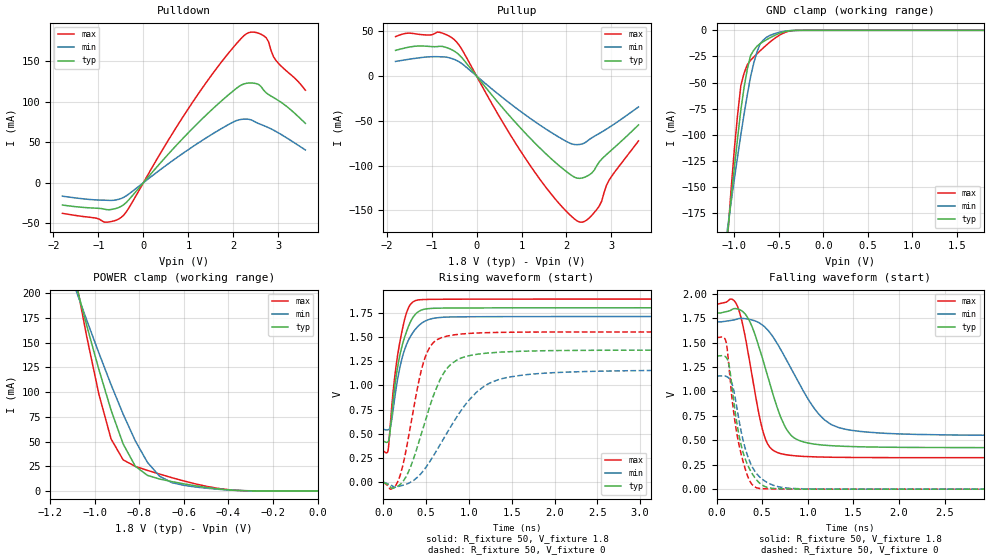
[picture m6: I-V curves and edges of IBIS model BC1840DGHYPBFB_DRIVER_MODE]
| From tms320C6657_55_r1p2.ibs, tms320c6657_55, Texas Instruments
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|   Model Cell BC1840DGHYPBFB_DRIVER_MODE
|BC1840DGHYPBFB_DRIVER_MODE
[Model]   BC1840DGHYPBFB_DRIVER_MODE
Model_type   I/O
Polarity   Non-Inverting
Enable   Active-Low
Vinl =  0.63
Vinh =  1.17
Cref = 5.0000pF
Rref =  100.0000M
Vref =  0V
Vmeas =  0.9
C_comp   1.10911p   1.03952p   1.18892p
[Model Spec]
Vinl   0.63   0.5985   0.6615
Vinh   1.17   1.1115   1.2285
D_overshoot_high 2.34 2.34 2.34
D_overshoot_low -0.3 -0.3 -0.3
D_overshoot_time 1.00E-09 1.00E-09 1.00E-09
S_overshoot_high 1.98 1.98 1.98
S_overshoot_low 0 0 0
[Temperature Range]   25   105   -40
[Voltage Range]   1.8   1.71   1.89
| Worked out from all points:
|   slope of the pulldown table from 0 to 0.27 V, typ, clamps not added: 15.4 ohm
|   slope of the pullup table from 0 to 0.27 V, typ, clamps not added: 15.9 ohm
|   GND clamp passes 1 mA (typ) near -0.42 V on its own axis
|   POWER clamp passes 1 mA (typ) near -0.40 V on its own axis
|   rising waveform, R_fixture 50, V_fixture 1.8: 20-80 % time 161ps typ, 181ps min, 137ps max; typ from 0.424 V to 1.8 V
|   rising waveform, R_fixture 50, V_fixture 0: 20-80 % time 317ps typ, 530ps min, 210ps max; typ from 0 V to 1.36 V
|   falling waveform, R_fixture 50, V_fixture 1.8: 20-80 % time 279ps typ, 437ps min, 186ps max; typ from 1.8 V to 0.424 V
|   falling waveform, R_fixture 50, V_fixture 0: 20-80 % time 165ps typ, 184ps min, 146ps max; typ from 1.36 V to 0 V
[POWER_clamp]
|   voltage   I(typ)   I(min)   I(max)
-1.8V     876.1mA    681mA      1.159A
-1.073V   198.5mA    195.8mA    199.1mA
-981.8mV  123mA      139.7mA    98mA
-927.3mV  81.99mA    107.7mA    52.77mA
-872.7mV  47.54mA    77.69mA    31.43mA
-818.2mV  25.01mA    50.7mA     24.89mA
-763.6mV  15.74mA    28.92mA    20.82mA
-709.1mV  12.03mA    14.9mA     17.05mA
-654.5mV  9.456mA    8.449mA    13.46mA
-490.9mV  3.25mA     2.59mA     4.308mA
-381.8mV  737.2uA    709.9uA    826.7uA
0V        21.76nA    38.43nA    32.18nA
[Pulldown]
|   voltage   I(typ)   I(min)   I(max)
-1.8V     -27.59mA   -16.63mA   -37.9mA
-818.2mV  -33.28mA   -21.71mA   -48.81mA
-600mV    -31.68mA   -21.18mA   -46.2mA
-436.4mV  -27.13mA   -18.06mA   -39.96mA
545.5mV   34.85mA    23.08mA    51.77mA
1.145V    70.05mA    46.38mA    103.7mA
1.964V    112mA      74.07mA    165mA
2.291V    122.9mA    78.62mA    184.1mA
2.564V    121.4mA    73.06mA    184.7mA
2.727V    111.2mA    69.38mA    179.4mA
2.945V    103.5mA    63.37mA    151.2mA
3.6V      73.39mA    40.47mA    114.4mA
[Pullup]
|   voltage   I(typ)   I(min)   I(max)
-1.8V     28.57mA    16.24mA    43.9mA
-872.7mV  32.76mA    21.51mA    48.97mA
-490.9mV  27.62mA    18.41mA    40.38mA
-327.3mV  20.49mA    13.81mA    29.81mA
490.9mV   -30.3mA    -20.58mA   -43.91mA
1.2V      -69.85mA   -47.55mA   -100.4mA
1.855V    -100.9mA   -68.97mA   -143.4mA
2.291V    -114.3mA   -76.45mA   -163mA
2.564V    -108.3mA   -68.99mA   -155.5mA
2.727V    -96.01mA   -64.18mA   -145.2mA
2.945V    -85.16mA   -57.48mA   -116.5mA
3.6V      -54.64mA   -34.55mA   -72.5mA
[GND_clamp]
|   voltage   I(typ)   I(min)   I(max)
-1.8V     -868mA     -670.8mA   -1.158A
-1.073V   -191.9mA   -187.1mA   -194.7mA
-1V       -131.4mA   -142.5mA   -113.9mA
-927.3mV  -76.42mA   -99.89mA   -52.96mA
-890.9mV  -54.65mA   -80.26mA   -41.03mA
-818.2mV  -24.17mA   -44.53mA   -28.69mA
-781.8mV  -18.98mA   -31.19mA   -25.53mA
-709.1mV  -12.66mA   -12.66mA   -19.47mA
-636.4mV  -8.859mA   -6.522mA   -13.85mA
-454.5mV  -1.754mA   -1.121mA   -2.894mA
-309.1mV  -64.58uA   -60.71uA   -100.3uA
1.8V      21.76nA    434.6nA    31.79nA
[Ramp]
| variable   typ   min   max
dV/dt_f   0.853734/0.28765375n   0.720228/0.44934898n   0.97377/0.1922822n
dV/dt_r  0.8551926/0.32908632n   0.725223/0.54823312n   0.973686/0.21779407n
R_load = 50
[Rising Waveform]
R_fixture = 50
V_fixture = 1.8
V_fixture_min = 1.71
V_fixture_max = 1.89
|   time   V(typ)   V(min)   V(max)
0s        424mV      546.4mV    321.1mV
56.26ps   419.6mV    541mV      335.4mV
89.4ps    623.2mV    601mV      694mV
133.2ps   987.6mV    874.4mV    1.096V
225.6ps   1.432V     1.304V     1.594V
292ps     1.606V     1.465V     1.798V
369.8ps   1.729V     1.574V     1.873V
521ps     1.791V     1.676V     1.887V
781.8ps   1.798V     1.705V     1.889V
4.992ns   1.8V       1.71V      1.89V
[Rising Waveform]
R_fixture = 50
V_fixture = 0
V_fixture_min = 0
V_fixture_max = 0
|   time   V(typ)   V(min)   V(max)
0s        0V         0V         0V
149.2ps   -49.05mV   -50.3mV    -25.82mV
259.5ps   47.54mV    -23.18mV   306.6mV
474.5ps   590.6mV    126.5mV    1.253V
562.2ps   836.1mV    239.7mV    1.418V
683.6ps   1.094V     418.9mV    1.493V
849.9ps   1.256V     662.8mV    1.523V
1.087ns   1.319V     926.6mV    1.539V
1.461ns   1.346V     1.083V     1.548V
4.992ns   1.363V     1.157V     1.551V
[Falling Waveform]
R_fixture = 50
V_fixture = 1.8
V_fixture_min = 1.71
V_fixture_max = 1.89
|   time   V(typ)   V(min)   V(max)
0s        1.801V     1.711V     1.89V
224.4ps   1.845V     1.74V      1.882V
351.7ps   1.739V     1.738V     1.367V
506.8ps   1.328V     1.676V     598.5mV
575.2ps   1.107V     1.613V     440.3mV
682.4ps   788.3mV    1.463V     369.5mV
879.2ps   509.3mV    1.125V     339.7mV
1.15ns    452.5mV    739.3mV    328.4mV
1.4ns     438.2mV    615.3mV    324.8mV
4.992ns   424.4mV    547.4mV    322mV
[Falling Waveform]
R_fixture = 50
V_fixture = 0
V_fixture_min = 0
V_fixture_max = 0
|   time   V(typ)   V(min)   V(max)
0s        1.362V     1.157V     1.551V
104.2ps   1.35V      1.154V     1.508V
139.1ps   1.261V     1.132V     1.221V
172ps     1.028V     1.071V     909.3mV
246.4ps   551.3mV    704.1mV    453.7mV
344.6ps   240mV      328.5mV    124.2mV
438.2ps   94.85mV    160.8mV    14.22mV
599.9ps   9.428mV    47.98mV    2.69mV
847.5ps   2.318mV    6.517mV    0V
4.992ns   0V         0V         0V
